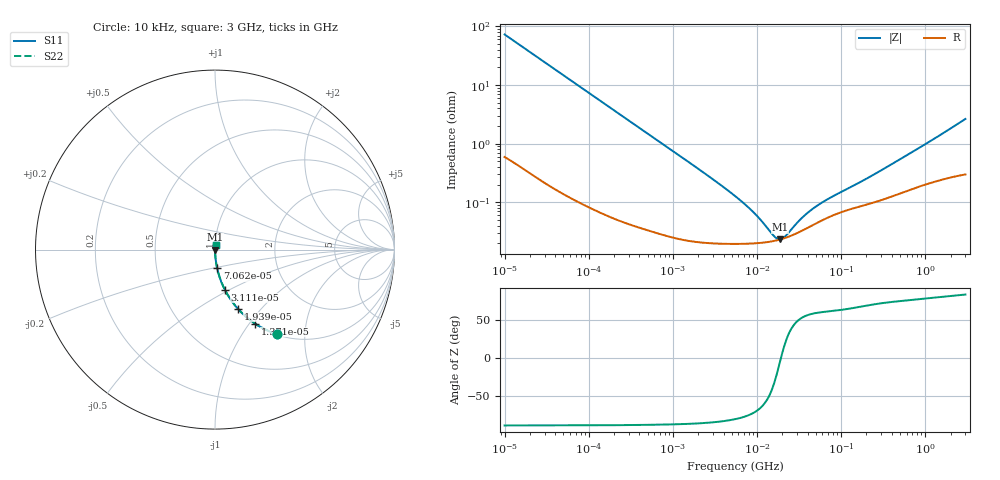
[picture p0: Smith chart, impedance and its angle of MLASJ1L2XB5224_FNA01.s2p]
! MLASJ1L2XB5224_FNA01  S-PARAMETER MODEL  ( Standard Model )
! Model Generated by TAIYO YUDEN Corporation (http://www.ty-top.com)
! Version 1.0
! TAIYO YUDEN Control No. 220601
! Copyright(c) 2010 TAIYO YUDEN CO.,LTD. All Rights Reserved.
! Product Description (link to TY-COMPAS)
! https://ds.yuden.co.jp/TYCOMPAS/or/detail?pn=MLASJ1L2XB5224KFNA01&u=M
! Products Name : Multilayer Ceramic Capacitors
! Characteristics :
!  Capacitance : 0.22 [uF] , Rated Voltage : 6.3 [V] , TCC : X5R
!  Case Size : 1.0 x 0.5 / 0.039 x 0.02 [mm/inch] , Thickness : 0.2 / 0.008 [mm/inch]
!  (Conditions: Temperature = 25 [degC] , DC Bias Voltage = 0 [V])
! External Node Assignments :
!  1  o---| |---o  2
! GND o---------o GND
! Frequency Range : 10kHz  -  3GHz  [ 401 STEP ]
# MHZ S RI R 50
! Freq[MHz].  S11 Real  S11 Imag  S21 Real  S21 Imag  S12 Real  S12 Imag  S22 Real  S22 Imag
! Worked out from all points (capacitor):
!   401 points, 10 kHz to 3 GHz, reference 50 ohm
!   read as one part in series: C = 218 nF near 10.65 kHz
!   lowest |Z| = 23.2 mohm at 18.73 MHz (marker M1)
!   series resonance near 19.3 MHz, so ESL is about 310 pH
!   S11 on the Smith chart (normalised r, x): 10 kHz: 1.01, -1.46; 13.71 kHz: 1.01, -1.07; 19.39 kHz: 1.01, -0.75; 31.11 kHz: 1.00, -0.47; 70.62 kHz: 1.00, -0.21; 3 GHz: 1.01, +0.05
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0.01  0.3482 -0.4724  0.6518 0.4724  0.6518 0.4724  0.3482 -0.4724
0.013707  0.2231 -0.4122  0.7769 0.4122  0.7769 0.4122  0.2231 -0.4122
0.019389  0.1268 -0.3286  0.8732 0.3286  0.8732 0.3286  0.1268 -0.3286
0.031113  0.0544 -0.2225  0.9456 0.2225  0.9456 0.2225  0.0544 -0.2225
0.070624  0.0118 -0.103  0.9882 0.103  0.9882 0.103  0.0118 -0.103
0.082683  0.0088 -0.0883  0.9912 0.0883  0.9912 0.0883  0.0088 -0.0883
0.199902  0.00189 -0.037  0.9981 0.037  0.9981 0.037  0.00189 -0.037
0.683653  0.000408 -0.0109  0.9996 0.0109  0.9996 0.0109  0.000408 -0.0109
2.570001  0.000209 -0.00287  0.9998 0.00287  0.9998 0.00287  0.000209 -0.00287
5.477226  0.000196 -0.00126  0.9998 0.00126  0.9998 0.00126  0.000196 -0.00126
9.361346  0.000199 -0.000613  0.9998 0.000613  0.9998 0.000613  0.000199 -0.000613
15.99985  0.000218 -0.000145  0.9998 0.000145  0.9998 0.000145  0.000218 -0.000145
17.5871  0.000225 -7.13e-05  0.9998 7.13e-05  0.9998 7.13e-05  0.000225 -7.13e-05
18.73182  0.00023 -2.28e-05  0.9998 2.28e-05  0.9998 2.28e-05  0.00023 -2.28e-05
19.95104  0.000237 2.52e-05  0.9998 -2.52e-05  0.9998 -2.52e-05  0.000237 2.52e-05
21.93027  0.000247 9.67e-05  0.9998 -9.67e-05  0.9998 -9.67e-05  0.000247 9.67e-05
33.04079  0.000318 0.000404  0.9997 -0.000404  0.9997 -0.000404  0.000318 0.000404
45.28751  0.000401 0.000644  0.9996 -0.000644  0.9996 -0.000644  0.000401 0.000644
70.41703  0.000551 0.001  0.9994 -0.001  0.9994 -0.001  0.000551 0.001
187.1348  0.000888 0.00222  0.9991 -0.00222  0.9991 -0.00222  0.000888 0.00222
374.4521  0.00122 0.00404  0.9988 -0.00404  0.9988 -0.00404  0.00122 0.00404
3000  0.00365 0.026  0.9964 -0.026  0.9964 -0.026  0.00365 0.026
